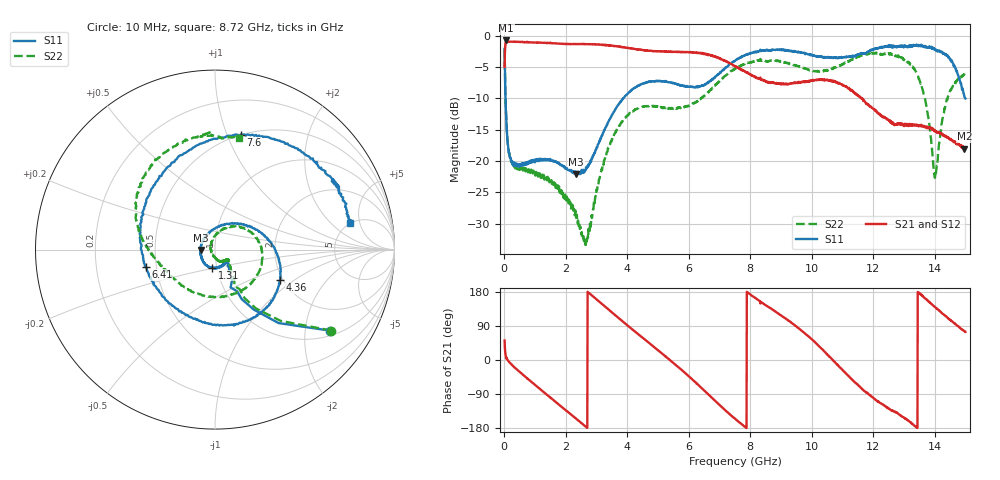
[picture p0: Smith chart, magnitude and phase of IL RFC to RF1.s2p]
!Agilent Technologies,N5230A,MY45001650,A.07.50.48
!Agilent N5230A: A.07.50.48
!Date: Wednesday, April 30, 2014 16:43:51
!Correction: S11(Full 2 Port(1,2))
!S21(Full 2 Port(1,2))
!S12(Full 2 Port(1,2))
!S22(Full 2 Port(1,2))
!S2P File: Measurements: S11, S21, S12, S22:
# Hz S  dB  R 50
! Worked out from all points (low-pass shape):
!   1500 points, 10 MHz to 15 GHz, reference 50 ohm
!   highest |S21| = -0.75 dB at 60 MHz (marker M1); lowest = -18.0 dB at 14.97 GHz (marker M2)
!   |S21| within 3 dB of the highest: 15.49 MHz to 7.04 GHz (7.024 GHz wide, 199 % of centre); 7.041384 GHz to 7.06414 GHz (22.76 MHz wide, 0.323 % of centre)
!   lowest |S11| = -22.1 dB at 2.34 GHz (marker M3), VSWR 1.17, Z = 42.7 - j0.118 ohm
!   |S11| at or under -10 dB: 39.55 MHz to 3.86 GHz (3.82 GHz wide, 196 % of centre); 3.862084 GHz to 3.872149 GHz (10.06 MHz wide, 0.26 % of centre); 14.99792 GHz to end of sweep
!   |S22| runs from -33.6 to -2.1 dB; largest |S21 - S12| = 0.015
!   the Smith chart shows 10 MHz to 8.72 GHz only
!   S11 on the Smith chart (normalised r, x): 10 MHz: 1.15, -2.73; 1.31 GHz: 0.95, -0.19; 4.36 GHz: 1.93, -0.79; 6.41 GHz: 0.44, -0.10; 7.6 GHz: 0.50, +1.12; 8.72 GHz: 4.98, +3.56
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1e7  -2.09 -35.1  -4.99 51.6  -4.97 51.4  -2.06 -34.8
6e7  -12.83 -67.6  -0.75 4.2  -0.77 4.1  -12.78 -61.9
2.8e8  -20.12 -43.9  -0.97 -15.7  -0.95 -15.7  -20.41 -38.3
1.31e9  -19.83 -99.5  -1.12 -86.6  -1.13 -86.6  -22.77 -63.8
2.34e9  -22.11 -179.0  -1.32 -155.0  -1.31 -155.1  -29.05 -106.6
2.51e9  -21.60 155.6  -1.32 -166.4  -1.32 -166.5  -31.58 -131.0
3.53e9  -12.40 32.0  -1.59 123.6  -1.60 123.7  -16.22 55.4
4.36e9  -7.94 -25.3  -2.16 67.9  -2.16 67.9  -11.55 -4.8
5.01e9  -7.19 -61.5  -2.49 25.3  -2.48 25.3  -11.32 -57.9
6.41e9  -7.99 -166.1  -2.82 -73.4  -2.79 -73.5  -9.98 -164.9
7.51e9  -3.97 84.3  -4.83 -155.5  -4.89 -155.2  -5.23 140.1
7.6e9  -3.65 77.5  -5.10 -161.3  -5.09 -161.1  -5.03 135.4
8.72e9  -2.30 11.0  -7.51 133.5  -7.52 133.3  -3.94 78.0
1.001e10  -3.08 -62.8  -7.11 54.1  -7.15 54.1  -5.63 -7.3
1.066e10  -3.56 -114.4  -7.32 2.0  -7.19 2.1  -5.23 -62.4
1.129e10  -3.25 -179.0  -8.65 -49.8  -8.76 -49.5  -3.82 -105.9
1.251e10  -1.80 79.3  -13.49 -128.3  -13.51 -128.0  -2.78 -153.0
1.349e10  -1.63 36.2  -14.44 177.9  -14.36 177.4  -6.91 171.4
1.402e10  -2.17 13.7  -15.28 139.2  -15.15 139.1  -22.15 61.4
1.452e10  -3.92 -19.5  -16.52 104.7  -16.49 104.5  -8.57 -39.4
1.497e10  -9.70 -97.5  -18.03 76.1  -18.02 76.4  -6.12 -44.7
1.5e10  -10.02 -107.5  -17.94 74.1  -17.87 74.3  -5.86 -44.0
